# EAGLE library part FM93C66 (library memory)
4096-Bit Serial CMOS EEPROM (MICROWIRE TM Synchronous Bus) Source: www.fairchildsemi.com
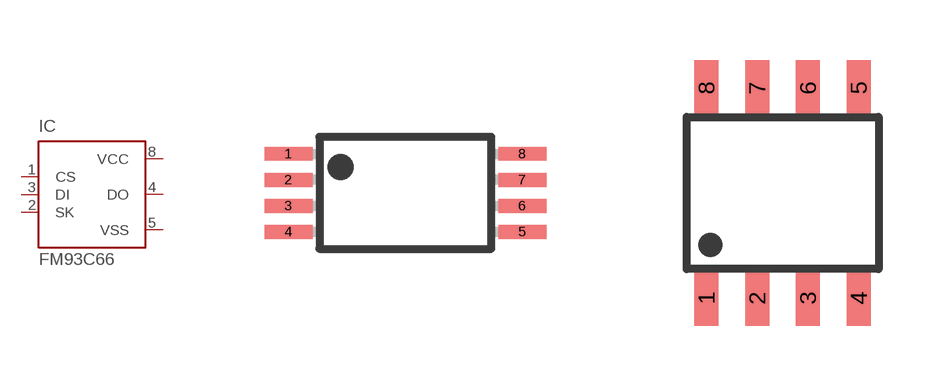
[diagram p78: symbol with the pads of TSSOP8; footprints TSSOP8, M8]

Designator prefix IC

## FM93C66MT8  [TSSOP8]
1  CS  in
2  SK  in
3  DI  in
4  DO  hiz
5  VSS  pwr
8  VCC  pwr

## FM93C66M  [M8]
Pads as for TSSOP8

## FM93C66N  [DIL08]
Pads as for TSSOP8

## Footprint TSSOP8 (pad centres in mm)
8-Pin Molded TSSOP, JEDEC (MT8) Package Number MTC08 Source: www.fairchildsemi.com
smd 1.2 x 0.35: 1 -2.925,0.975; 2 -2.925,0.325; 3 -2.925,-0.325; 4 -2.925,-0.975; 5 2.925,-0.975; 6 2.925,-0.325; 7 2.925,0.325; 8 2.925,0.975

## Footprint M8 (pad centres in mm)
Molded Package, Small Outline, 0.15 Wide, 8-Lead (M8) Package Number M08A Source: www.fairchildsemi.com
smd 0.6 x 1.4: 1 -1.905,-2.63; 2 -0.635,-2.63; 3 0.635,-2.63; 4 1.905,-2.63; 5 1.905,2.63; 6 0.635,2.63; 7 -0.635,2.63; 8 -1.905,2.63

## Footprint DIL08 (pad centres in mm)
Dual In Line Package
drill 0.813 long: 1 -3.81,-3.81; 2 -1.27,-3.81; 3 1.27,-3.81; 4 3.81,-3.81; 5 3.81,3.81; 6 1.27,3.81; 7 -1.27,3.81; 8 -3.81,3.81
